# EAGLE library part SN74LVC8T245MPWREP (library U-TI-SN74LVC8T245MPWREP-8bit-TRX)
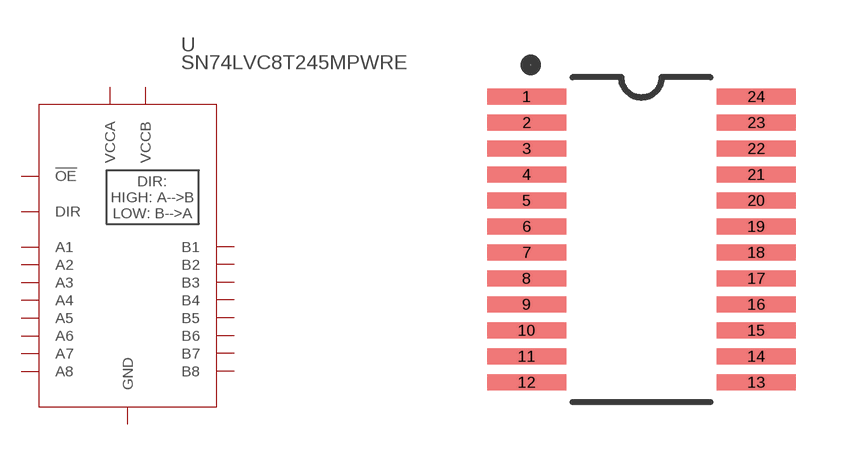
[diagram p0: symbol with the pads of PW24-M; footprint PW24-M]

Designator prefix U

## SN74LVC8T245MPWREPPW24-M (MANUFACTURER_PART_NUMBER: SN74LVC8T245MPWREP; VENDOR: Texas Instruments)  [PW24-M]
1  VCCA  pwr
2  DIR  in
3  A1
4  A2
5  A3
6  A4
7  A5
8  A6
9  A7
10  A8
11  GND  pwr
12  GND  pwr
13  GND  pwr
14  B8
15  B7
16  B6
17  B5
18  B4
19  B3
20  B2
21  B1
22  !OE  in
23  VCCB  pwr
24  VCCB  pwr

## Footprint PW24-M (pad centres in mm)
smd 1.981 x 0.406: 1 -2.87,3.575; 2 -2.87,2.925; 3 -2.87,2.275; 4 -2.87,1.625; 5 -2.87,0.975; 6 -2.87,0.325; 7 -2.87,-0.325; 8 -2.87,-0.975; 9 -2.87,-1.625; 10 -2.87,-2.275; 11 -2.87,-2.925; 12 -2.87,-3.575; 13 2.87,-3.575; 14 2.87,-2.925; 15 2.87,-2.275; 16 2.87,-1.625; 17 2.87,-0.975; 18 2.87,-0.325; 19 2.87,0.325; 20 2.87,0.975; 21 2.87,1.625; 22 2.87,2.275; 23 2.87,2.925; 24 2.87,3.575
